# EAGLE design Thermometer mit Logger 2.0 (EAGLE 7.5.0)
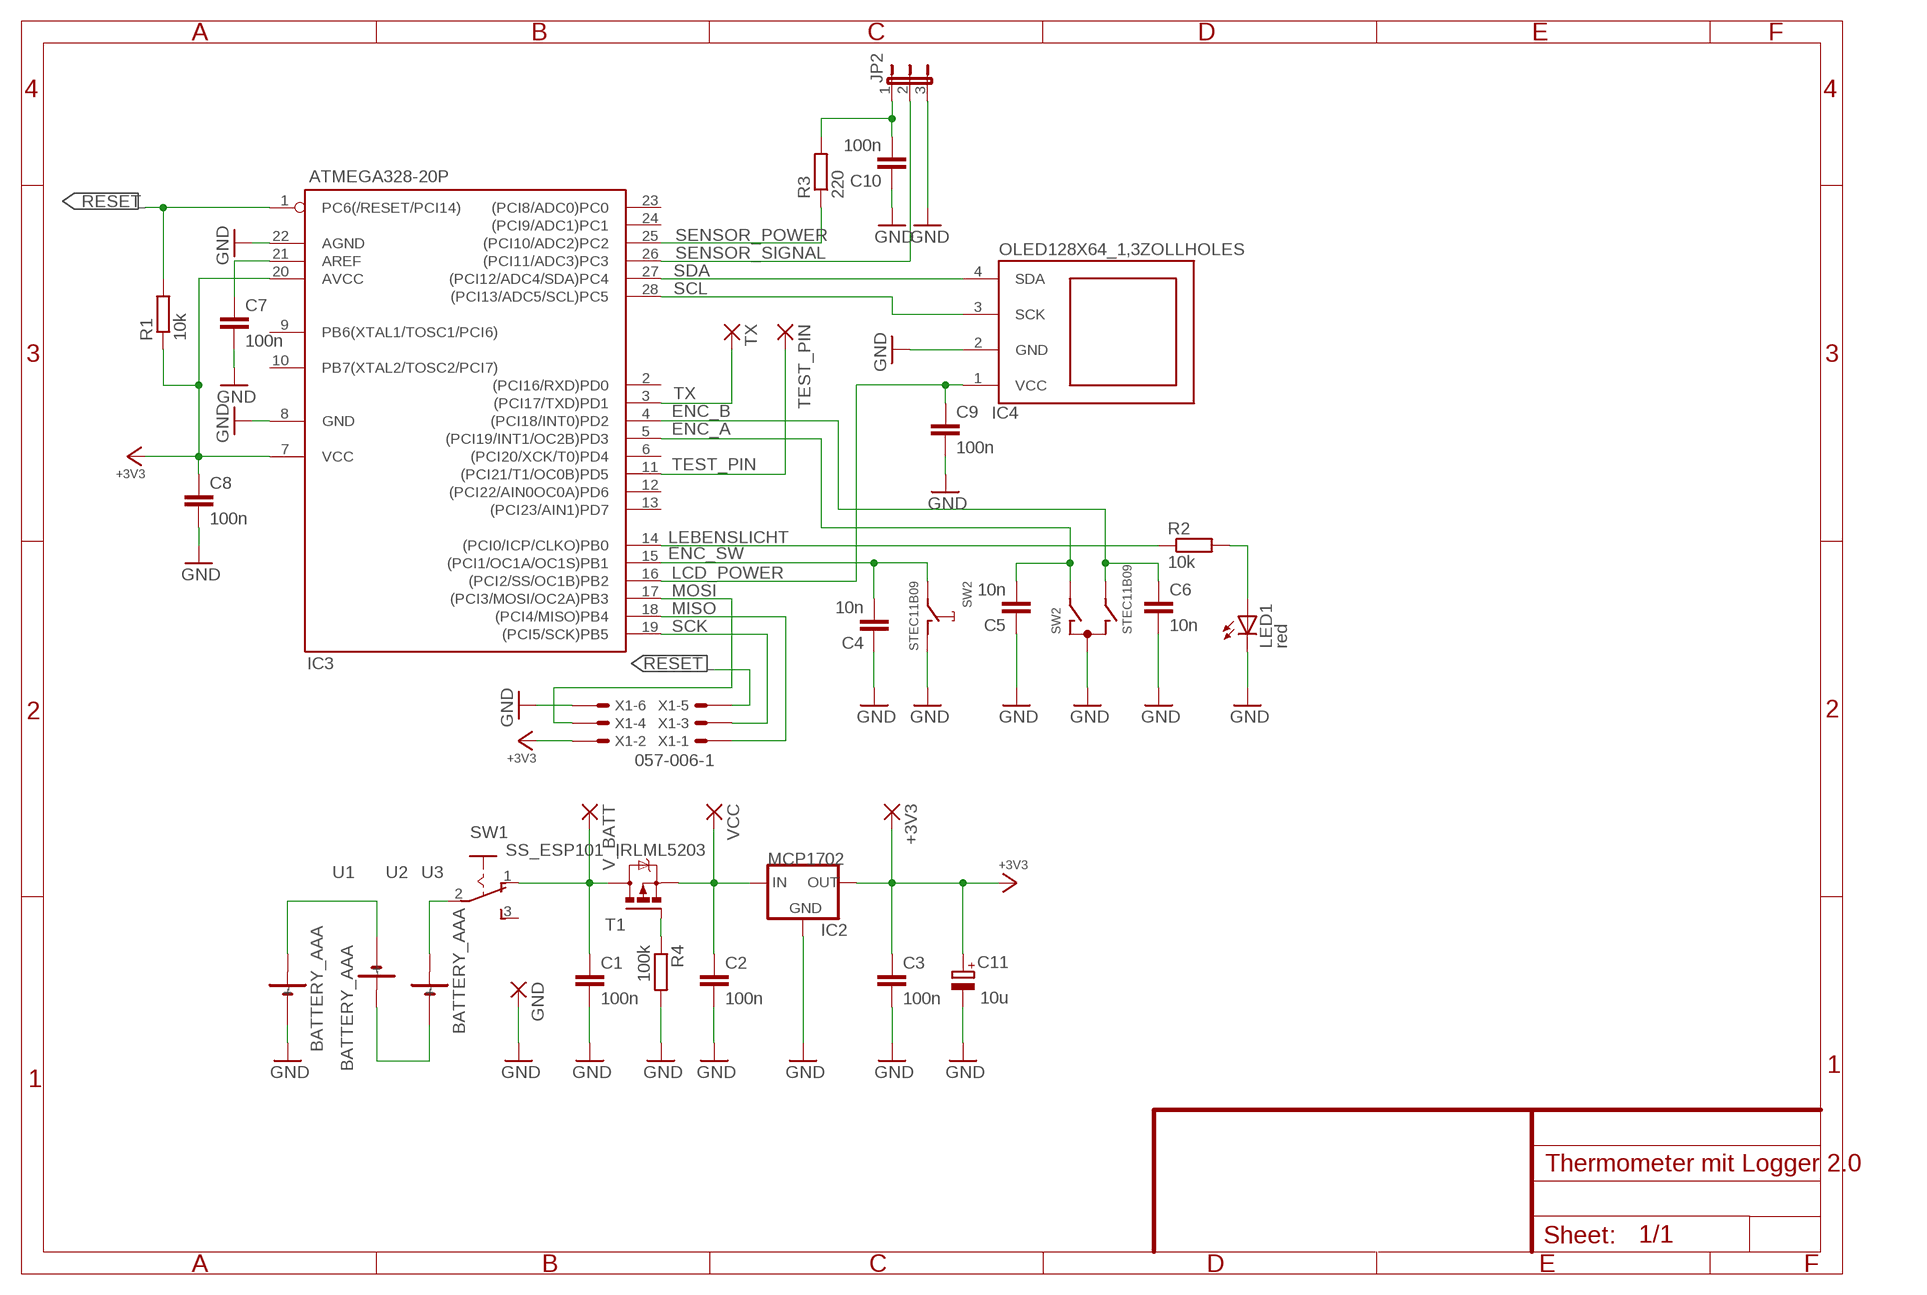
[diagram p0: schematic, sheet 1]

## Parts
+3V3  +3V3  2,15/1,0  [2,15/1,0]
C1  100n  C-EU025-024X044  [C025-024X044]
C2  100n  C-EU025-024X044  [C025-024X044]
C3  100n  C-EU025-024X044  [C025-024X044]
C4  10n  C-EU025-024X044  [C025-024X044]
C5  10n  C-EU025-024X044  [C025-024X044]
C6  10n  C-EU025-024X044  [C025-024X044]
C7  100n  C-EU025-024X044  [C025-024X044]
C8  100n  C-EU025-024X044  [C025-024X044]
C9  100n  C-EU025-024X044  [C025-024X044]
C10  100n  C-EU025-024X044  [C025-024X044]
C11  10u  CPOL-EUE1.8-4  [E1,8-4]
GND  GND  2,15/1,0  [2,15/1,0]
IC2  MCP1702  [TO92]
IC3  ATMEGA328-20P  ATMEGA168-20P  [DIL28-3]
IC4  OLED128X64_1,3ZOLLHOLES  [OLED128X64_1,3ZOLL]
JP2  JP2E  [JP2]
LED1  red  LED3MM  [LED3MM]
R1  10k  R-EU_0207/10  [0207/10]
R2  10k  R-EU_0207/10  [0207/10]
R3  220  R-EU_0207/10  [0207/10]
R4  100k  R-EU_0207/10  [0207/10]
SW1  SS_ESP101  [SS_ESP101]
SW2  STEC11B09  INKREMENTAL_ENCODERSTEC11B09  [STEC11B09]
T1  IRLML5203  [MICRO3]
TEST_PIN  TEST_PIN  2,15/1,0  [2,15/1,0]
TX  TX  2,15/1,0  [2,15/1,0]
U1  BATTERY_AAA  [BATTERY_HOLDER_AAA_KEYSTONE]
U2  BATTERY_AAA  [BATTERY_HOLDER_AAA_KEYSTONE]
U3  BATTERY_AAA  [BATTERY_HOLDER_AAA_KEYSTONE]
V_BATT  V_BATT  2,15/1,0  [2,15/1,0]
VCC  VCC  2,15/1,0  [2,15/1,0]
X1  057-006-1  [057-006-1]

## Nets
+3V3: +3V3.1(P) C3.1 C8.1 C11.+ IC2.3(OUT) IC3.7(VCC) IC3.20(AVCC) R1.1 X1.2
ENC_A: C5.2 IC3.5((PCI19/INT1/OC2B)PD3) SW2.A(E:A)
ENC_B: C6.1 IC3.4((PCI18/INT0)PD2) SW2.B(E:B)
ENC_SW: C4.2 IC3.15((PCI1/OC1A/OC1S)PB1) SW2.E
GND: C1.2 C2.2 C3.2 C4.1 C5.1 C6.2 C7.2 C8.2 C9.2 C10.1 C11.- GND.1(P) IC2.1(GND) IC3.8(GND) IC3.22(AGND) IC4.2(GND) JP2.3 LED1.K(C) R4.2 SW2.C(E:C) SW2.D U1.P$2(-) X1.6
LCD_POWER: C9.1 IC3.16((PCI2/SS/OC1B)PB2) IC4.1(VCC)
LEBENSLICHT: IC3.14((PCI0/ICP/CLKO)PB0) R2.1
MISO: IC3.18((PCI4/MISO)PB4) X1.1
MOSI: IC3.17((PCI3/MOSI/OC2A)PB3) X1.4
N$2: R4.1 T1.1(G)
N$3: C7.1 IC3.21(AREF)
N$5: U1.P$1(+) U2.P$2(-)
N$6: U2.P$1(+) U3.P$2(-)
N$7: C10.2 JP2.1 R3.2
N$8: SW1.2(P) U3.P$1(+)
N$15: LED1.A R2.2
RESET: IC3.1(PC6(/RESET/PCI14)) R1.2 X1.5
SCK: IC3.19((PCI5/SCK)PB5) X1.3
SCL: IC3.28((PCI13/ADC5/SCL)PC5) IC4.3(SCK)
SDA: IC3.27((PCI12/ADC4/SDA)PC4) IC4.4(SDA)
SENSOR_POWER: IC3.25((PCI10/ADC2)PC2) R3.1
SENSOR_SIGNAL: IC3.26((PCI11/ADC3)PC3) JP2.2
TEST_PIN: IC3.11((PCI21/T1/OC0B)PD5) TEST_PIN.1(P)
TX: IC3.3((PCI17/TXD)PD1) TX.1(P)
V_BATT: C1.1 SW1.1(O) T1.3(D) V_BATT.1(P)
VCC: C2.1 IC2.2(IN) T1.2(S) VCC.1(P)
Unconnected: IC3.2((PCI16/RXD)PD0) IC3.6((PCI20/XCK/T0)PD4) IC3.9(PB6(XTAL1/TOSC1/PCI6)) IC3.10(PB7(XTAL2/TOSC2/PCI7)) IC3.12((PCI22/AIN0OC0A)PD6) IC3.13((PCI23/AIN1)PD7) IC3.23((PCI8/ADC0)PC0) IC3.24((PCI9/ADC1)PC1) SW1.3(S) SW2.GND1(G) SW2.GND2(G)

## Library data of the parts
+3V3 GND TEST_PIN TX V_BATT VCC = wirepad:2,15/1,0: THROUGH-HOLE PAD
C1-C10 = rcl:C-EU: CAPACITOR, European symbol
C11 = rcl:CPOL-EU: POLARIZED CAPACITOR, European symbol
IC2 = TEWE:MCP1702
IC3 = avr:ATMEGA168*P: MICROCONTROLLER 16 kBytes FLASH 1 kBytes SRAM 512 Bytes EEPROM USART 8-channel 10 bit ADC
IC4 = AAN1_V1R01:OLED128X64_1,3ZOLL
JP2 = jumper:JP2E: JUMPER
LED1 = led:LED: LED
R1-R4 = rcl:R-EU_: RESISTOR, European symbol
SW1 = TEWE:SS_ESP101
SW2 = AAN1_V1R01:INKREMENTAL_ENCODER: ALPS rotary Encoder EC12E series with switch
T1 = transistor-power:IRLML5203: HEXFET P-Channel Power MOSFET
U1-U3 = TEWE:BATTERY_AAA
X1 = con-panduit:057-006-: CONNECTOR 6-pin series 057 contact pc board low profile headers

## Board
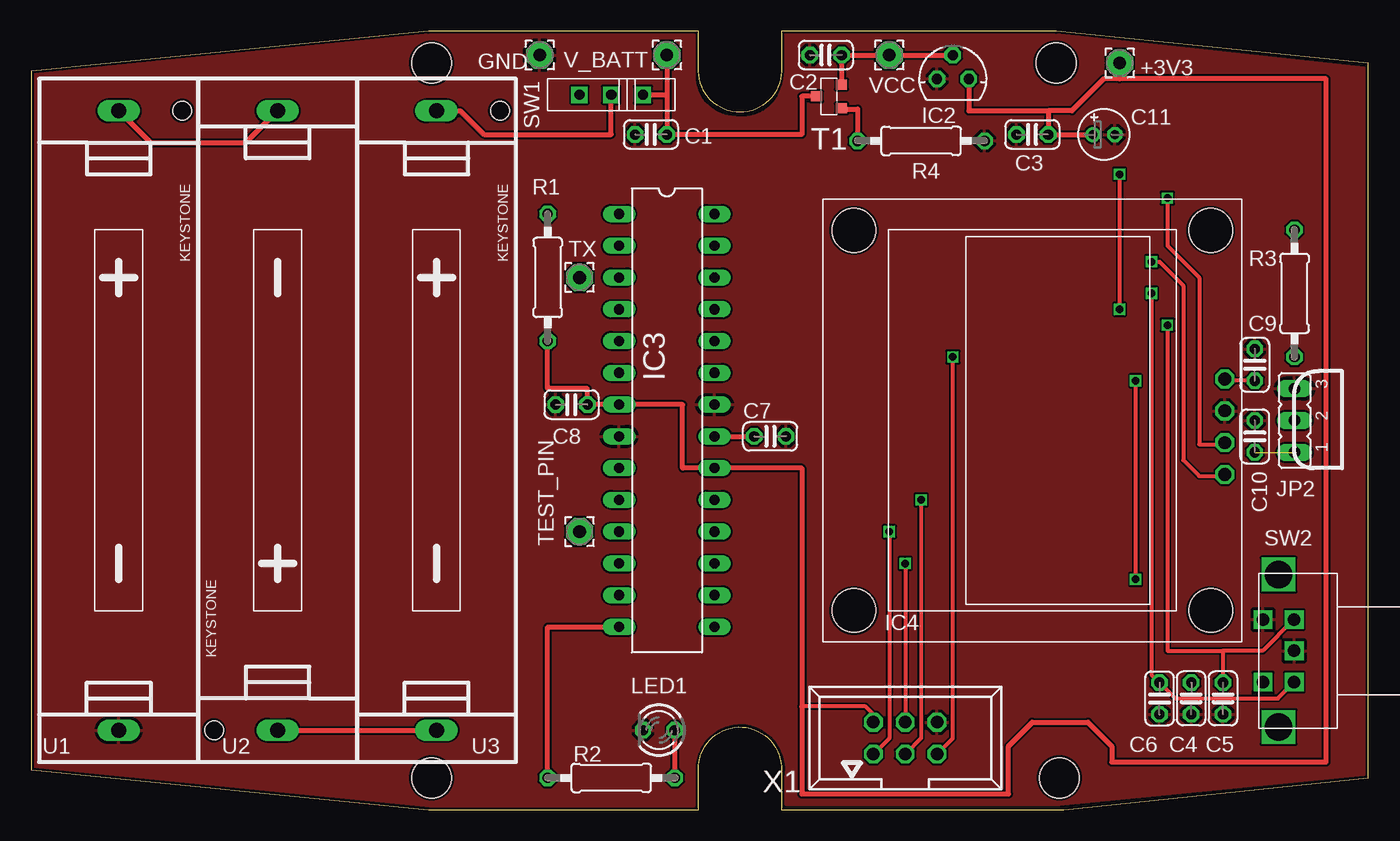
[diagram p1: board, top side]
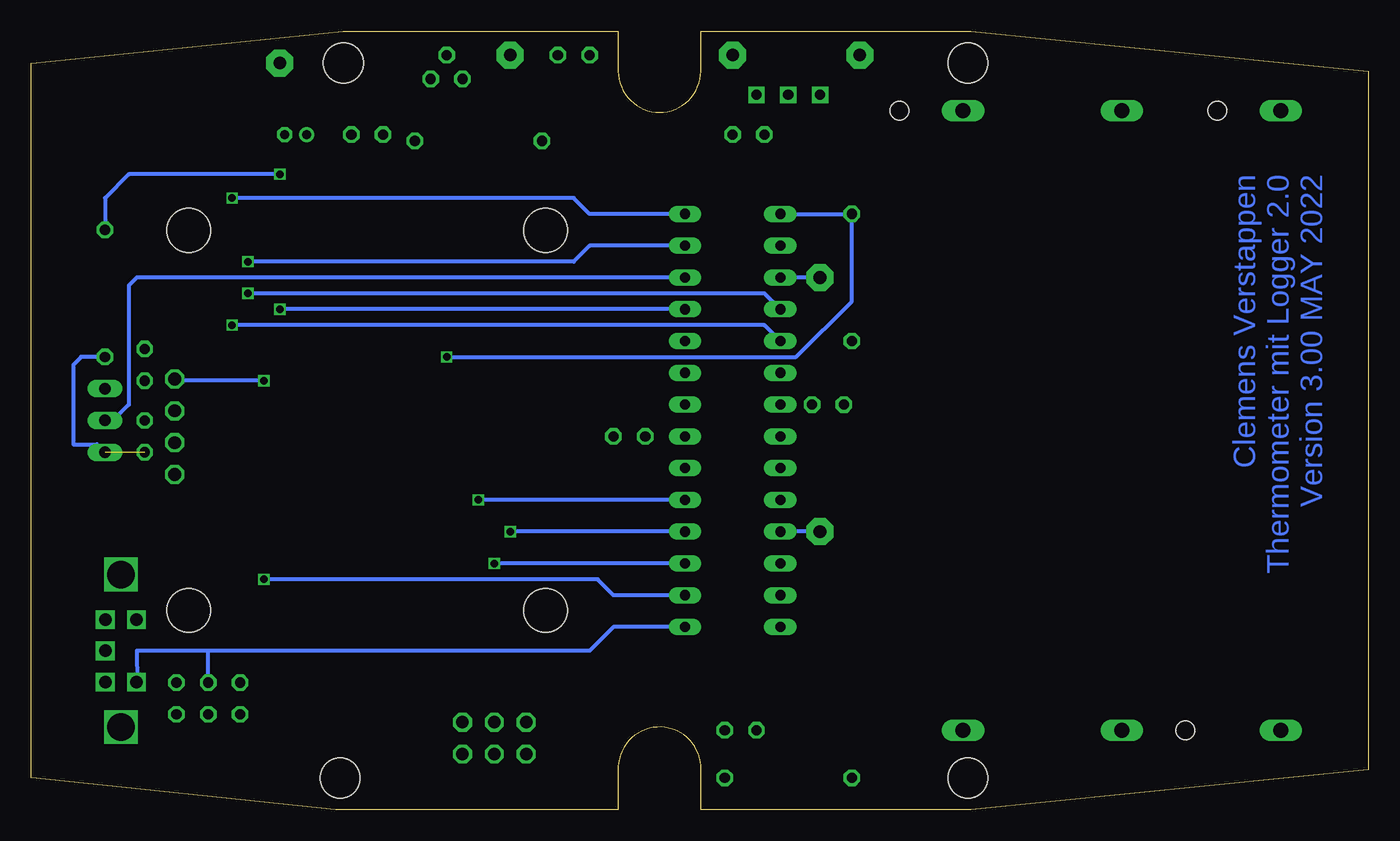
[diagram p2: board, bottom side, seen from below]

Size 106.86 x 62.23 mm. Coordinates in mm from the lower left corner, seen from the top.
Outline: 0,3.17 31.75,0 53.34,0 53.34,3.17 arc-180 59.94,3.43 59.94,0 82.55,0 106.86,2.54 106.86,59.68 81.92,62.23 59.94,62.23 59.94,59.05 arc-180 53.34,59.05 53.34,62.23 31.75,62.23 0,59.05 0,3.17
Copper layers (1*16): Top 0.035mm / dielectric 1.5mm / Bottom 0.035mm
Design rules "aisler_2_layer": minimum track width 0.1mm, minimum drill 0.2mm, track to track 0.15mm, track to pad 0.1mm, pad to pad 0.1mm, via to via 0.1mm, smd to smd 0.1mm, copper to edge 0.2mm, drill to drill 0.21mm, minimum pad ring 0.25mm, minimum via ring 0.15mm, stop-mask expansion 0mil, vias tented up to drill 0mil, thermal gap 10mil
Holes 3.2 mm at 32,2.54 82.17,2.54 32,59.69 81.92,59.69

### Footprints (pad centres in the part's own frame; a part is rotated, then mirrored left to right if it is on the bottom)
2,15/1,0 = drill 1.016 pad 2.159 octagon: 1 0,0
C025-024X044 = drill 0.813 octagon: 1 -1.27,0; 2 1.27,0
E1,8-4 = drill 0.711 pad 1.168: + -0.889,0 | drill 0.711 pad 1.168 octagon: - 0.889,0
TO92 = drill 0.813 octagon: 1 -1.27,0; 2 0,1.905; 3 1.27,0
DIL28-3 = drill 0.813 long: 1 -16.51,-3.81; 2 -13.97,-3.81; 3 -11.43,-3.81; 4 -8.89,-3.81; 5 -6.35,-3.81; 6 -3.81,-3.81; 7 -1.27,-3.81; 8 1.27,-3.81; 9 3.81,-3.81; 10 6.35,-3.81; 11 8.89,-3.81; 12 11.43,-3.81; 13 13.97,-3.81; 14 16.51,-3.81; 15 16.51,3.81; 16 13.97,3.81; 17 11.43,3.81; 18 8.89,3.81; 19 6.35,3.81; 20 3.81,3.81; 21 1.27,3.81; 22 -1.27,3.81; 23 -3.81,3.81; 24 -6.35,3.81; 25 -8.89,3.81; 26 -11.43,3.81; 27 -13.97,3.81; 28 -16.51,3.81
OLED128X64_1,3ZOLL = drill 1.016 octagon: 1 -3.31,15.385; 2 -0.77,15.385; 3 1.77,15.385; 4 4.31,15.385 | hole 3.5: -15.2,-14.25; 15.2,-14.25; 15.2,14.25; -15.2,14.25
JP2 = drill 0.914 long: 1 -2.54,0; 2 0,0; 3 2.54,0
LED3MM = drill 0.813 octagon: A -1.27,0; K 1.27,0
0207/10 = drill 0.813 octagon: 1 -5.08,0; 2 5.08,0
SS_ESP101 = drill 0.813 square: 1 -2.54,0; 2 0,0; 3 2.54,0
STEC11B09 = drill 1 square: A -2.5,1.25; B 2.5,1.25; C 0,1.25; D -2.5,-1.25; E 2.5,-1.25 | drill 2.2 square: GND1 -6.1,0; GND2 6.1,0
MICRO3 = smd 0.8 x 0.9: 1 -0.95,-1; 2 0.95,-1; 3 0,1
BATTERY_HOLDER_AAA_KEYSTONE = drill 1.2 long: P$1 52.07,6.35; P$2 2.54,6.35 | hole 1.5: 52.07,1.27
057-006-1 = drill 1 octagon: 1 -2.54,-1.27; 2 -2.54,1.27; 3 0,-1.27; 4 0,1.27; 5 2.54,-1.27; 6 2.54,1.27

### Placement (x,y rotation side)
+3V3  87,59.69 0 top
C1  49.53,53.98 180 top
C2  63.5,60.32 180 top
C3  80.01,53.98 180 top
C4  92.71,8.89 90 top
C5  95.25,8.89 90 top
C6  90.17,8.89 270 top
C7  59.05,29.84 0 top
C8  43.18,32.38 180 top
C9  97.79,35.56 90 top
C10  97.79,29.84 270 top
C11  85.72,53.98 0 top
GND  40.64,60.32 0 top
IC2  73.66,58.42 0 top
IC3  50.8,31.11 270 top
IC4  80.01,31.11 270 top
JP2  100.97,31.11 90 top
LED1  50.16,6.35 180 top
R1  41.27,42.55 90 top
R2  46.35,2.54 0 top
R3  100.97,41.27 270 top
R4  71.12,53.47 0 top
SW1  46.35,57.15 180 top
SW2  99.69,12.7 270 top
T1  63.75,57.02 90 top
TEST_PIN  43.81,22.22 0 top
TX  43.81,42.55 0 top
U1  13.34,3.81 90 top
U2  13.34,58.42 270 top
U3  38.73,3.81 90 top
V_BATT  50.8,60.32 0 top
VCC  68.58,60.32 0 top
X1  69.85,5.71 0 top

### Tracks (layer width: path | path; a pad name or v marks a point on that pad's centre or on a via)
+3V3
  Top 0.305: X1.2 67.31,7.62 66.67,8.25 61.59,8.25
  Top 0.406: 87,58.42 103.5,58.42 103.5,3.81 86.36,3.81 86.36,5.08 84.45,6.99 80.01,6.99 78.11,5.08 78.11,1.27 61.59,1.27 61.59,8.25 61.59,27.3 IC3.20 52.07,27.3 52.07,32.38 IC3.7 C8.1 44.45,33.66 41.27,33.66 R1.1 | IC2.3 74.93,55.88 81.28,55.88 | 81.28,55.88 C3.1 C11.+ | +3V3.1 87,58.42 | 87,58.42 85.72,58.42 83.19,55.88 81.28,55.88
ENC_A  (via drill 0.6)
  Top 0.305: v90.81,38.73 90.81,12.7 95.25,12.7 | 95.25,12.7 C5.2 | SW2.A 100.92,15.2 98.42,12.7 95.25,12.7
  Bottom 0.305: IC3.5 48.26,38.73 v90.81,38.73
ENC_B  (via drill 0.6)
  Top 0.305: v89.53,41.27 89.53,10.8 C6.1 91.44,8.89 99.64,8.89 SW2.B
  Bottom 0.305: IC3.4 48.26,41.27 v89.53,41.27
ENC_SW
  Bottom 0.305: IC3.15 60.33,14.61 62.23,12.7 92.71,12.7 | C4.2 92.71,12.7 | 92.71,12.7 98.42,12.7 98.41,10.16 SW2.E
GND
  pour Top: 0.25,3.43 0.25,58.8 31.5,61.98 52.96,61.98 52.96,58.67 arc90 56.26,55.37 arc104 60.2,58.93 60.2,61.98 81.92,61.98 106.55,59.31 106.55,2.79 82.17,0.38 60.33,0.38 60.33,2.54 arc191 52.96,3.17 52.96,0.25 31.88,0.25
LCD_POWER  (via drill 0.6)
  Top 0.305: v88.27,18.41 v88.27,34.29 | C9.1 95.53,34.29
  Top 0.406: 95.53,34.29 IC4.1
  Bottom 0.305: IC3.16 60.33,17.14 61.59,18.41 v88.27,18.41 | v88.27,34.29 95.26,34.29
  Bottom 0.406: 95.26,34.29 IC4.1
LEBENSLICHT
  Top 0.406: R2.1 41.27,14.61 IC3.14
MISO  (via drill 0.6)
  Top 0.305: v68.58,22.22 68.58,5.71 X1.1
  Bottom 0.305: IC3.18 v68.58,22.22
MOSI  (via drill 0.6)
  Top 0.305: v69.85,19.68 X1.4
  Bottom 0.305: IC3.17 v69.85,19.68
N$2
  Top 0.406: T1.1 64.82,56.01 66.04,56.01 R4.1
N$3
  Top 0.406: IC3.21 C7.1
N$5
  Top 0.406: U1.P$1 9.53,53.34 17.14,53.34 U2.P$2
N$6
  Top 0.406: U2.P$1 U3.P$2
N$7  (1 unrouted)
  Bottom 0.305: R3.2 102.87,36.2 103.5,35.56 103.5,29.21 101.6,29.21 JP2.1
N$8
  Top 0.406: U3.P$1 34.29,55.88 36.2,53.98 46.35,53.98 SW1.2
N$15
  Top 0.406: R2.2 LED1.A
RESET  (via drill 0.6)
  Top 0.305: v73.66,36.2 73.66,5.71 X1.5
  Bottom 0.305: IC3.1 R1.2 41.27,40.64 45.72,36.2 v73.66,36.2
SCK  (via drill 0.6)
  Top 0.305: v71.12,24.77 71.12,5.71 X1.3
  Bottom 0.305: IC3.19 v71.12,24.77
SCL  (via drill 0.6)
  Top 0.305: v90.81,48.89 90.81,45.09 93.34,42.55 93.34,29.21 95.26,29.21 IC4.3
  Bottom 0.305: IC3.28 62.23,47.62 63.5,48.89 v90.81,48.89
SDA  (via drill 0.6)
  Top 0.305: v89.53,43.81 90.17,43.81 92.08,41.91 92.08,27.94 93.34,26.67 95.26,26.67 IC4.4
  Bottom 0.305: IC3.27 62.23,45.09 63.5,43.81 v89.53,43.81
SENSOR_POWER  (via drill 0.6)
  Top 0.305: v87,40.01 v87,50.8
  Bottom 0.305: IC3.25 v87,40.01 | v87,50.8 99.06,50.8 100.97,48.89 R3.1
SENSOR_SIGNAL
  Bottom 0.305: IC3.26 98.42,42.55 99.06,41.91 99.06,32.38 100.33,31.11 JP2.2
TEST_PIN
  Bottom 0.305: TEST_PIN.1 IC3.11
TX
  Bottom 0.305: TX.1 IC3.3
V_BATT
  Top 0.406: SW1.1 50.8,57.15 | V_BATT.1 50.8,57.15 | 50.8,57.15 C1.1 61.59,53.98 61.59,57.02 T1.3
VCC
  Top 0.406: T1.2 C2.1 VCC.1 IC2.2

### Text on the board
Bottom: Clemens Verstappen / Thermometer mit Logger 2.0 / Version 3.00 MAY 2022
